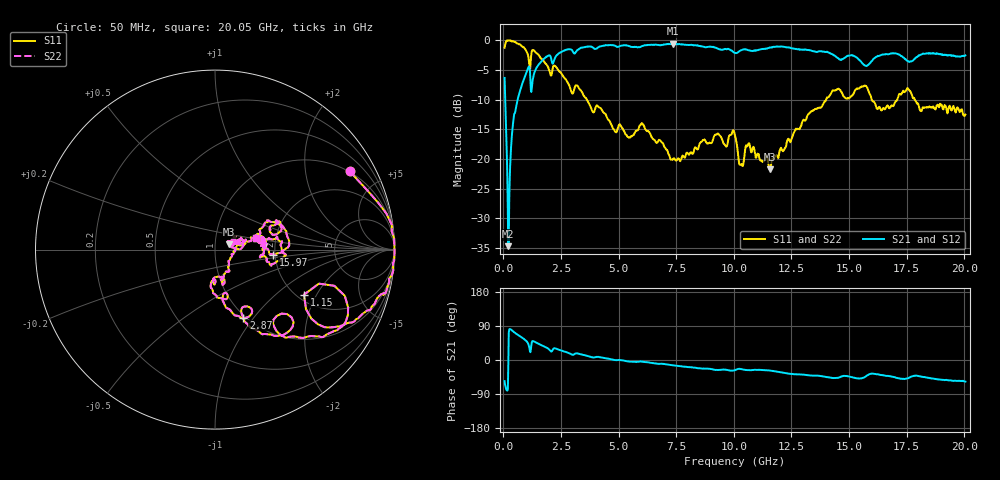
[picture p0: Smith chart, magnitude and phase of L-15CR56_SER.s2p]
! P/N: L-15CR56JE
! Measured by Marlon
! Oct. 13, 2003
! Measure with Series-through-Fixture
#	mhz	s	ma	r	50
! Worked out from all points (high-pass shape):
!   1001 points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, 50 MHz to 20.05 GHz, reference 50 ohm
!   highest |S21| = -0.56 dB at 7.35 GHz (marker M1); lowest = -34.7 dB at 210 MHz (marker M2)
!   |S21| within 3 dB of the highest: 2.178 GHz to 15.52 GHz (13.34 GHz wide, 151 % of centre); 17.65 GHz to end of sweep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
!   lowest |S11| = -21.8 dB at 11.55 GHz (marker M3), VSWR 1.18, Z = 58.2 + j3.35 ohm
!   |S11| at or under -10 dB: 3.619 GHz to 14 GHz (10.38 GHz wide, 118 % of centre); 15.99 GHz to 17.09 GHz (1.101 GHz wide, 6.65 % of centre); 17.85 GHz to end of sweep
!   |S22| runs from -21.8 to 0.0 dB; largest |S21 - S12| = 0
!   S11 on the Smith chart (normalised r, x): 50 MHz: 0.98, +3.45; 1.15 GHz: 2.18, -1.58; 2.87 GHz: 0.97, -0.89; 15.97 GHz: 1.95, -0.12; 20.05 GHz: 1.57, +0.21
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50  0.8676 30.2  0.4828 -55.7  0.4828 -55.7  0.8676 30.2
210  1 -0.1  0.01836 -17.1  0.01836 -17.1  1 -0.1
290  0.9968 -5.3  0.08664 81.7  0.08664 81.7  0.9968 -5.3
530  0.964 -14.8  0.2619 70.1  0.2619 70.1  0.964 -14.8
970  0.8276 -30.6  0.5204 51.4  0.5204 51.4  0.8276 -30.6
1150  0.5556 -26.9  0.555 23.0  0.555 23.0  0.5556 -26.9
1570  0.7327 -41.2  0.6387 41.3  0.6387 41.3  0.7327 -41.2
2870  0.4106 -67.4  0.8449 17.3  0.8449 17.3  0.4106 -67.4
3390  0.3714 -74.3  0.8683 14.7  0.8683 14.7  0.3714 -74.3
4830  0.1718 -94.2  0.9045 -0.1  0.9045 -0.1  0.1718 -94.2
6730  0.1435 -59.5  0.9167 -10.0  0.9167 -10.0  0.1435 -59.5
7350  0.09886 -38.8  0.9374 -14.0  0.9374 -14.0  0.09886 -38.8
10050  0.157 6.5  0.788 -26.7  0.788 -26.7  0.157 6.5
10310  0.08968 23.9  0.8264 -24.1  0.8264 -24.1  0.08968 23.9
10610  0.1313 33.6  0.8285 -26.8  0.8285 -26.8  0.1313 33.6
11550  0.0817 20.5  0.873 -27.6  0.873 -27.6  0.0817 20.5
13390  0.2531 20.5  0.8157 -41.2  0.8157 -41.2  0.2531 20.5
15350  0.3935 23.2  0.7127 -48.3  0.7127 -48.3  0.3935 23.2
15970  0.3236 -4.9  0.6683 -36.1  0.6683 -36.1  0.3236 -4.9
16730  0.2695 11.8  0.7688 -42.7  0.7688 -42.7  0.2695 11.8
17550  0.3944 -5.0  0.6717 -48.1  0.6717 -48.1  0.3944 -5.0
20050  0.2366 15.5  0.7474 -57.0  0.7474 -57.0  0.2366 15.5
